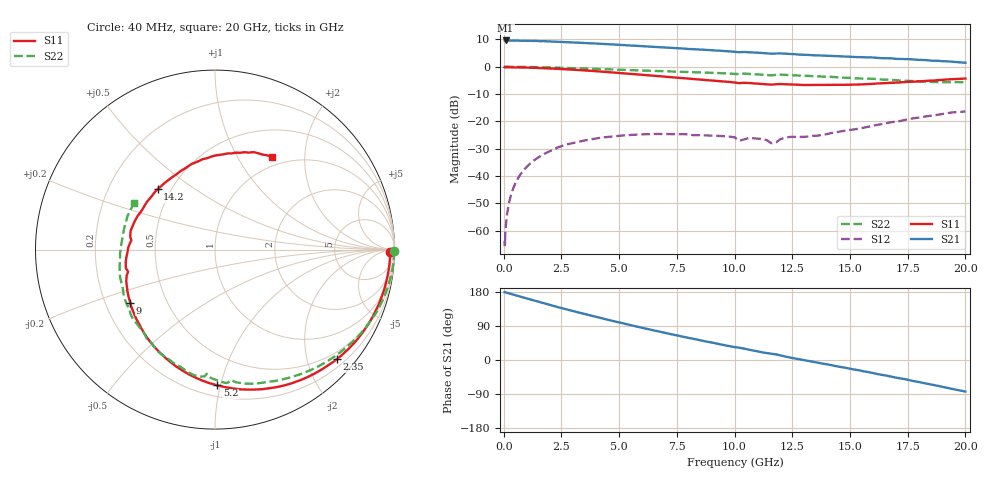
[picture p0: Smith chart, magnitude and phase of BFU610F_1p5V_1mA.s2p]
! Filename:  P:\Prog\Test\Noise\ATS_data\Testdata_Net\SplitFiles\BFU610_2W_A5_HighFreq_1.5V_1mA_D.s2p
! Date/Time: Wed 10/Aug/2011 16:53:57
! BFU610_2W_A5_HighFreq_Bias1_1.5V_1mA_10mA_R.s2p
! MDIF S-parameter v. bias file
! BFU610_2W_A5_HighFreq_1.5V_1mA_10mA
! Date/time Mon Aug 08 13:57:57 2011
! bias mode 1
! bias variable = I_out
! VAR bias_var= 1
! VAR V_out= 1.5001
! VAR I_out= 0.9950
! VAR V_in= 0.8498
! VAR I_in= 0.0074
! Device data file deembeded for feedlines and parallel
! Original file: \SplitFiles\BFU610_2W_A5_HighFreq_1.5V_1mA_R.s2p
! Feed-files: PR003V01_101208_Feed1.s2p, PR003V01_101208_Feed2.s2p
! Parallel-file: PR003V01_101208_Par.s2p
# MHz S MA R 50
!  Freq-MHz  S11-mag  S11-arg  S21-mag  S21-arg  S12-mag  S12-arg  S22-mag  S22-arg
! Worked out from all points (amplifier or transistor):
!   167 points, 40 MHz to 20 GHz, reference 50 ohm
!   highest |S21| = 9.6 dB at 80 MHz (marker M1)
!   |S21| within 3 dB of that: start of sweep to 7.847 GHz
!   unconditionally stable (mu >= 1): 7.8 GHz to end of sweep
!   at 550 MHz: K = -0.01, MSG = 25.7 dB, |S12| = -41.9 dB
!   at 4.2 GHz: K = 0.42, MSG = 17.2 dB, |S12| = -26.0 dB
!   at 20 GHz: K = 1.19, MAG = 6.2 dB, |S12| = -16.4 dB
!   S11 on the Smith chart (normalised r, x): 40 MHz: 65, -35; 2.35 GHz: 0.35, -2.56; 5.2 GHz: 0.28, -0.98; 9 GHz: 0.31, -0.26; 14.2 GHz: 0.42, +0.36; 20 GHz: 0.86, +1.41
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40  0.9765 -0.7  3.009 179.3  0.0005214 88.7  0.9976 -0.4
50  0.9707 -0.7  2.997 179.4  0.0006469 48.2  0.9979 -0.5
60  0.9792 -0.9  3.004 178.6  0.0005608 94.1  0.9982 -0.6
80  0.9763 -1.4  3.015 178.5  0.00104 90.7  0.9982 -0.8
140  0.9762 -2.5  3.002 177.5  0.001902 91.5  0.9979 -1.4
280  0.9751 -5.0  2.999 174.9  0.003964 90.1  0.9973 -2.8
700  0.969 -12.7  2.98 167.6  0.01031 83.7  0.9932 -7.1
1350  0.9522 -24.4  2.963 156.3  0.01981 74.0  0.9827 -13.5
2350  0.9126 -42.0  2.858 139.6  0.03361 61.2  0.9583 -23.0
3400  0.8598 -59.7  2.72 122.9  0.04379 47.3  0.9285 -32.3
4300  0.8091 -74.6  2.61 109.3  0.0506 37.4  0.9013 -39.7
5200  0.7564 -89.0  2.478 96.3  0.05538 28.5  0.8741 -46.9
6800  0.6645 -114.2  2.265 74.1  0.05872 14.6  0.8282 -59.1
7800  0.6122 -129.8  2.143 61.0  0.05819 7.9  0.8014 -66.4
9000  0.5568 -148.0  2 46.2  0.05483 3.1  0.7731 -75.2
10200  0.4991 -165.8  1.837 32.4  0.0441 -4.3  0.7325 -82.7
12000  0.4814 167.4  1.744 11.8  0.04748 17.4  0.7141 -97.1
13400  0.4632 145.0  1.619 -4.7  0.05432 16.1  0.6694 -110.9
14200  0.4652 133.3  1.575 -13.7  0.06116 20.0  0.6509 -119.0
16800  0.5085 97.8  1.421 -44.1  0.0965 15.0  0.5733 -151.3
18400  0.5524 78.0  1.306 -63.6  0.125 3.7  0.5294 -177.6
20000  0.607 58.4  1.179 -83.3  0.1521 -12.1  0.521 150.4
